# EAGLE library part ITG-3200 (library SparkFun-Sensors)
Invensense ITG-3200 3-Axis Gyroscope The ITG-3200 is the world’s first single-chip, digital-output, 3-axis MEMS motion processing gyro optimized for gaming, 3D mice, and motion-based remote control applications for Internet connected Digital TVs and Set Top Boxes. The ITG-3200 features three 16-bit analog-to-digital converters (ADCs) for digitizing the gyro outputs, a user-selectable internal low-pass filter bandwidth, and a Fast-Mode I²C (400kHz) interface. Additional features include an embedded temperature sensor and a 2% accurate internal oscillator. This breakthrough in MEMS motion processing gyro technology provides a dramatic 60% package size reduction, delivers a 60% power reduction, and has inherent cost advantages compared to competing multi-chip gyro solutions. Datasheet SparkFun Products Triple-Axis Digital-Output Gyroscope - ITG-3200 (SEN-09793) SparkFun Triple-Axis Digital-Output Gyro Breakout - ITG-3200 (SEN-11977) SparkFun 9 Degrees of Freedom - Sensor Stick (SEN-10724) SparkFun 6 Degrees of Freedom IMU Digital Combo Board - ITG3200/ADXL345 (SEN-10121) 9 Degrees of Freedom - Razor IMU (SEN-10736)
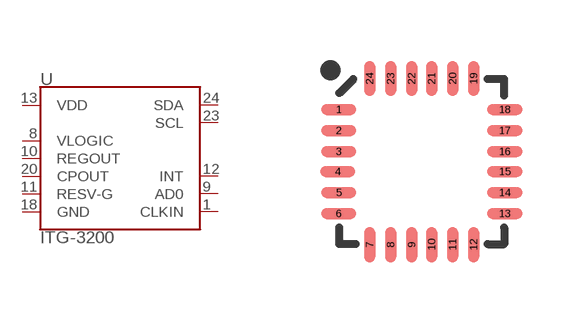
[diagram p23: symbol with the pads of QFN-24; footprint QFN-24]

Designator prefix U

## ITG-3200 (PROD_ID: IC-09685; SF_ID: SEN-09793)  [QFN-24]
1  CLKIN
8  VLOGIC
9  AD0
10  REGOUT
11  RESV-G
12  INT
13  VDD
18  GND
20  CPOUT
23  SCL
24  SDA

## Footprint QFN-24 (pad centres in mm)
24-Pin QFN (4 x 4 mm) (1:1 footprint) Datasheet Specifications: Pin Count: 24 Area: 4.0 x 4.0 x 0.9 mm Pitch: 0.5 mm Devices Using: ITG-3200
smd 0.889 x 0.279: 1 -2.076,1.301; 2 -2.076,0.775; 3 -2.076,0.25; 4 -2.102,-0.25; 5 -2.076,-0.775; 6 -2.076,-1.301; 13 2.076,-1.301; 14 2.076,-0.775; 15 2.076,-0.25; 16 2.076,0.25; 17 2.076,0.775; 18 2.076,1.301
smd 0.279 x 0.889: 7 -1.301,-2.076; 8 -0.775,-2.076; 9 -0.25,-2.076; 10 0.25,-2.076; 11 0.775,-2.076; 12 1.301,-2.076; 19 1.301,2.076; 20 0.775,2.076; 21 0.25,2.076; 22 -0.25,2.076; 23 -0.775,2.076; 24 -1.301,2.076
